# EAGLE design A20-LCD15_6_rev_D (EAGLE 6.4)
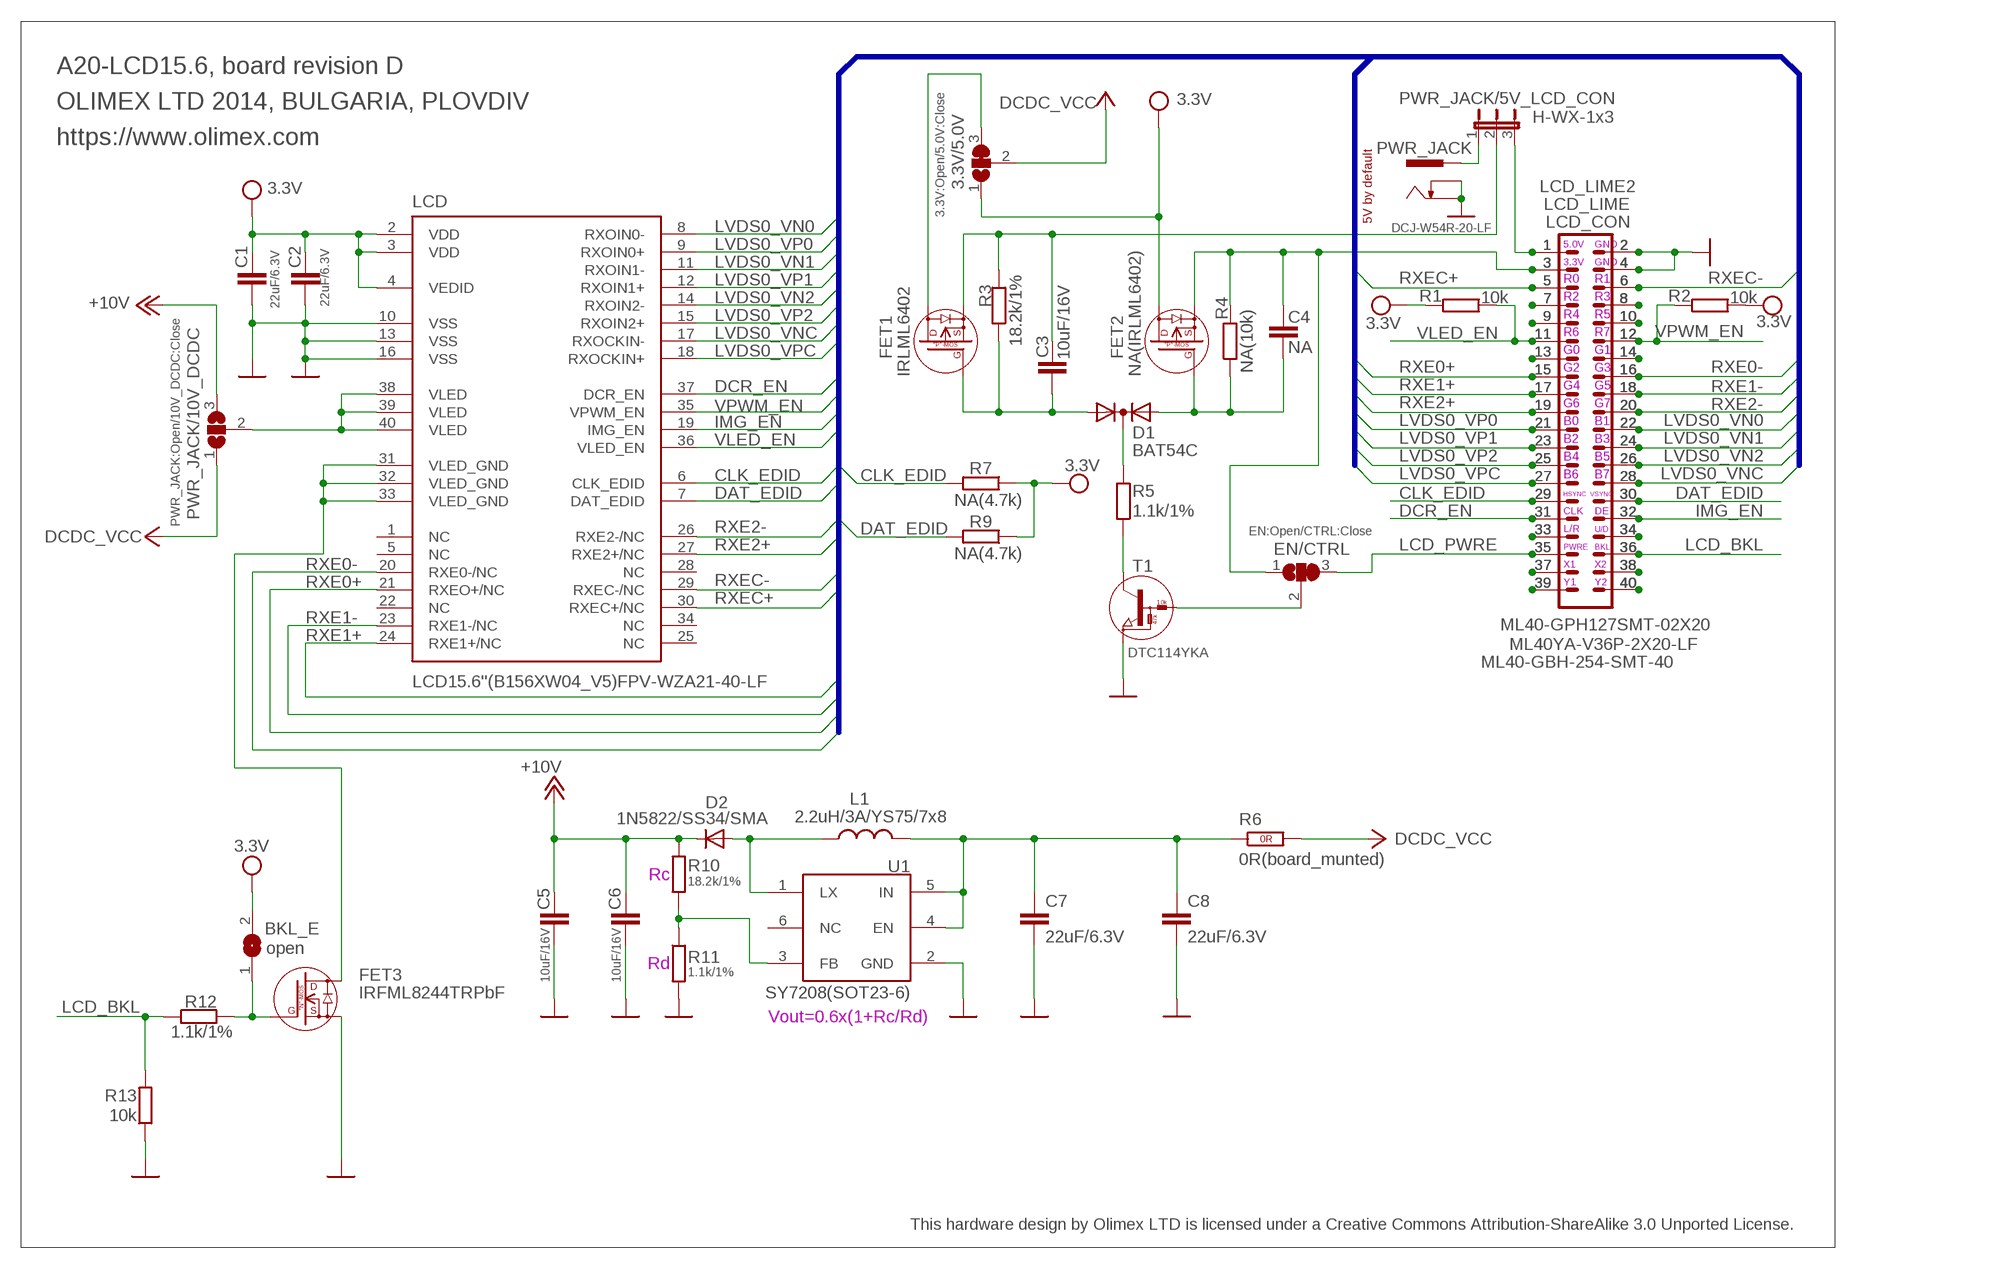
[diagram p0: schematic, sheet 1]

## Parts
3.3V/5.0V  3.3V:Open/5.0V:Close  SJ2W5  [SJ_2_SMALL_23_TIED]
BKL_E  open  SJSJ_1_THE_SMALLEST  [SJ_1_THE_SMALLEST]
C1  22uF/6.3V  C-EUC0603_DWS  [C0603_DWS]
C2  22uF/6.3V  C-EUC0603_DWS  [C0603_DWS]
C3  10uF/16V  C-EUC0805_5MIL_DWS  [C0805_5MIL_DWS]
C4  NA  C-EUC0603_DWS  [C0603_DWS]
C5  10uF/16V  C-EUC0805_5MIL_DWS  [C0805_5MIL_DWS]
C6  10uF/16V  C-EUC0805_5MIL_DWS  [C0805_5MIL_DWS]
C7  22uF/6.3V  C-EUC0805_5MIL_DWS  [C0805_5MIL_DWS]
C8  22uF/6.3V  C-EUC0805_5MIL_DWS  [C0805_5MIL_DWS]
D1  BAT54C  DIODE_AC-CA_  [SOT23C]
D2  1N5822/SS34/SMA  D-MLL-41  [MELF-MLL41]
EN/CTRL  EN:Open/CTRL:Close  SJ2W5  [SJ_2_SMALL_23_TIED]
FET1  IRLML6402  P-MOS+DIODIRLML6402  [SOT23]
FET2  NA(IRLML6402)  P-MOS+DIODIRLML6402  [SOT23]
FET3  IRFML8244TRPbF  N-MOS+DIODBSS138(SOT23-3)  [SOT23]
L1  2.2uH/3A/YS75/7x8  LLQH88PN100M38  [8X8MM_3131]
LCD  LCD15.6''(B156XW04_V5)FPV-WZA21-40-LF  [LCD_15.6'']
LCD_CON  ML40-GBH-254-SMT-40  [ML40-MALE(GBH-254-SMT-40)]
LCD_LIME  ML40YA-V36P-2X20-LF  [YA-V36P-2X20-LF]
LCD_LIME2  ML40-GPH127SMT-02X20  ML40-GPH127SMT-02X20(PA-V16X-2X20-LF)  [GPH127SMT-02X20(PA-V16X-2X20-LF)]
PWR_JACK  DCJ-W54R-20-LF  PWR-JAKDCJ-W  [PWR-JACK-SMD]
PWR_JACK/5V_LCD_CON  H-WX-1x3  JP2EHN1X3-SMD  [HN1X3-SMD]
PWR_JACK/10V_DCDC  PWR_JACK:Open/10V_DCDC:Close  SJ2W3  [SJ_2_SMALL]
R1  10k  R-EU_R0603_5MIL_DWS  [R0603_5MIL_DWS]
R2  10k  R-EU_R0603_5MIL_DWS  [R0603_5MIL_DWS]
R3  18.2k/1%  R-EU_R0603_5MIL_DWS  [R0603_5MIL_DWS]
R4  NA(10k)  R-EU_R0603_5MIL_DWS  [R0603_5MIL_DWS]
R5  1.1k/1%  R-EU_R0603_5MIL_DWS  [R0603_5MIL_DWS]
R6  0R(board_munted)  R_0R0R(NA)  [0603_0R]
R7  NA(4.7k)  R-EU_R0603_5MIL_DWS  [R0603_5MIL_DWS]
R9  NA(4.7k)  R-EU_R0603_5MIL_DWS  [R0603_5MIL_DWS]
R10  18.2k/1%  R-EU_R0603_5MIL_DWS  [R0603_5MIL_DWS]
R11  1.1k/1%  R-EU_R0603_5MIL_DWS  [R0603_5MIL_DWS]
R12  1.1k/1%  R-EU_R0603_5MIL_DWS  [R0603_5MIL_DWS]
R13  10k  R-EU_R0603_5MIL_DWS  [R0603_5MIL_DWS]
T1  DTC114YKA  DIGITAL_TRANSISTORS-NPNDTC114YKA  [SOT-23]
U1  SY7208(SOT23-6)  SY7208  [SOT23-6]

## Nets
3.3VDC [pwr]: C4.1 EN/CTRL.1 FET2.2(S) LCD_CON.3 LCD_LIME2.3 LCD_LIME.3 R4.2
5VDC: C3.1 FET1.2(S) PWR_JACK/5V_LCD_CON.2 R3.2
+5V: 3.3V/5.0V.2 PWR_JACK/10V_DCDC.1 R6.2(1.2) ; supply symbol labelled DCDC_VCC
+12V [pwr]: C5.1 C6.1 D2.1(C) PWR_JACK/10V_DCDC.3 R10.2 ; supply symbol labelled +10V
CLK_EDID: LCD.6(CLK_EDID) LCD_CON.29 LCD_LIME2.29 LCD_LIME.29 R7.2
DAT_EDID: LCD.7(DAT_EDID) LCD_CON.30 LCD_LIME2.30 LCD_LIME.30 R9.2
DCR_EN: LCD.37(DCR_EN) LCD_CON.31 LCD_LIME2.31 LCD_LIME.31
GND [pwr]: C1.2 C2.2 C5.2 C6.2 C7.2 C8.2 FET3.2(S) LCD.10(VSS) LCD.13(VSS) LCD.16(VSS) LCD_CON.2 LCD_CON.4 LCD_LIME2.2 LCD_LIME2.4 LCD_LIME.2 LCD_LIME.4 PWR_JACK.2(-) PWR_JACK.3(--) R11.2 R13.1 T1.2(E) U1.2(GND)
IMG_EN: LCD.19(IMG_EN) LCD_CON.32 LCD_LIME2.32 LCD_LIME.32
LCD_BKL: LCD_CON.36 LCD_LIME2.36 LCD_LIME.36 R12.1 R13.2
LCD_PWRE: EN/CTRL.3 LCD_CON.35 LCD_LIME2.35 LCD_LIME.35
LVDS0_VN0: LCD.8(RXOIN0-) LCD_CON.22 LCD_LIME2.22 LCD_LIME.22
LVDS0_VN1: LCD.11(RXOIN1-) LCD_CON.24 LCD_LIME2.24 LCD_LIME.24
LVDS0_VN2: LCD.14(RXOIN2-) LCD_CON.26 LCD_LIME2.26 LCD_LIME.26
LVDS0_VNC: LCD.17(RXOCKIN-) LCD_CON.28 LCD_LIME2.28 LCD_LIME.28
LVDS0_VP0: LCD.9(RXOIN0+) LCD_CON.21 LCD_LIME2.21 LCD_LIME.21
LVDS0_VP1: LCD.12(RXOIN1+) LCD_CON.23 LCD_LIME2.23 LCD_LIME.23
LVDS0_VP2: LCD.15(RXOIN2+) LCD_CON.25 LCD_LIME2.25 LCD_LIME.25
LVDS0_VPC: LCD.18(RXOCKIN+) LCD_CON.27 LCD_LIME2.27 LCD_LIME.27
N$1: 3.3V/5.0V.3 FET1.3(D)
N$2 [pwr]: FET3.3(D) LCD.31(VLED_GND) LCD.32(VLED_GND) LCD.33(VLED_GND)
N$3 [pwr]: LCD.38(VLED) LCD.39(VLED) LCD.40(VLED) PWR_JACK/10V_DCDC.2
N$4: BKL_E.1 FET3.1(G) R12.2
N$5: LCD_CON.7 LCD_LIME2.7 LCD_LIME.7
N$6: LCD_CON.9 LCD_LIME2.9 LCD_LIME.9
N$7: LCD_CON.13 LCD_LIME2.13 LCD_LIME.13
N$8: C4.2 D1.1(A1) FET2.1(G) R4.1
N$9: C3.2 D1.2(A2) FET1.1(G) R3.1
N$10: LCD_CON.33 LCD_LIME2.33 LCD_LIME.33
N$11: R5.1 T1.3(C)
N$12: LCD_CON.37 LCD_LIME2.37 LCD_LIME.37
N$13: LCD_CON.39 LCD_LIME2.39 LCD_LIME.39
N$14: LCD_CON.8 LCD_LIME2.8 LCD_LIME.8
N$15: LCD_CON.10 LCD_LIME2.10 LCD_LIME.10
N$16: EN/CTRL.2 T1.1(B)
N$17: LCD_CON.14 LCD_LIME2.14 LCD_LIME.14
N$18: LCD_CON.34 LCD_LIME2.34 LCD_LIME.34
N$19: D1.3(K) R5.2
N$20: LCD_CON.1 LCD_LIME2.1 LCD_LIME.1 PWR_JACK/5V_LCD_CON.3
N$21: LCD_CON.38 LCD_LIME2.38 LCD_LIME.38
N$22 [pwr]: PWR_JACK.1(+) PWR_JACK/5V_LCD_CON.1
N$23: LCD_CON.40 LCD_LIME2.40 LCD_LIME.40
N$24: C7.1 C8.1 L1.2 R6.1(1.1) U1.4(EN) U1.5(IN)
N$123: D2.2(A) L1.1 U1.1(LX)
N$126: R10.1 R11.1 U1.3(FB)
RXE0+: LCD.21(RXEO+/NC) LCD_CON.15 LCD_LIME2.15 LCD_LIME.15
RXE0-: LCD.20(RXE0-/NC) LCD_CON.16 LCD_LIME2.16 LCD_LIME.16
RXE1+: LCD.24(RXE1+/NC) LCD_CON.17 LCD_LIME2.17 LCD_LIME.17
RXE1-: LCD.23(RXE1-/NC) LCD_CON.18 LCD_LIME2.18 LCD_LIME.18
RXE2+: LCD.27(RXE2+/NC) LCD_CON.19 LCD_LIME2.19 LCD_LIME.19
RXE2-: LCD.26(RXE2-/NC) LCD_CON.20 LCD_LIME2.20 LCD_LIME.20
RXEC+: LCD.30(RXEC+/NC) LCD_CON.5 LCD_LIME2.5 LCD_LIME.5
RXEC-: LCD.29(RXEC-/NC) LCD_CON.6 LCD_LIME2.6 LCD_LIME.6
VCC [pwr]: 3.3V/5.0V.1 BKL_E.2 C1.1 C2.1 FET2.3(D) LCD.2(VDD) LCD.3(VDD) LCD.4(VEDID) R1.2 R2.1 R7.1 R9.1 ; supply symbol labelled 3.3V
VLED_EN: LCD.36(VLED_EN) LCD_CON.11 LCD_LIME2.11 LCD_LIME.11 R1.1
VPWM_EN: LCD.35(VPWM_EN) LCD_CON.12 LCD_LIME2.12 LCD_LIME.12 R2.2
Unconnected: LCD.1(NC) LCD.5(NC) LCD.22(NC) LCD.25(NC) LCD.28(NC) LCD.34(NC) U1.6(NC)

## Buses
LVDS0_VP[0..2],LVDS0_VN[0..2],LVDS0_VPC,LVDS0_VNC,CLK_EDID,DAT_EDID,DCR_EN,IMG_EN,VPWM_EN,VLED_EN,RXE0-,RXE0+,RXE1-,RXE1+,RXE2-,RXE2+,RXEC-,RXEC+

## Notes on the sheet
- A20-LCD15.6, board revision D
- OLIMEX LTD 2014, BULGARIA, PLOVDIV
- https://www.olimex.com
- 5V by default
- 5.0V | GND
- 3.3V | GND
- R0 | R1
- R2 | R3
- R4 | R5
- R6 | R7
- G0 | G1
- G2 | G3
- G4 | G5
- G6 | G7
- B0 | B1
- B2 | B3
- B4 | B5
- B6 | B7
- HSYNC | VSYNC
- CLK | DE
- L/R | U/D
- PWRE | BKL
- X1 | X2
- Y1 | Y2
- Rc
- Rd
- Vout=0.6x(1+Rc/Rd)
- This hardware design by Olimex LTD is licensed under a Creative Commons Attribution-ShareAlike 3.0 Unported License.

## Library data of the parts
3.3V/5.0V EN/CTRL PWR_JACK/10V_DCDC = jumper:SJ2W: SMD solder JUMPER
BKL_E = jumper:SJ: SMD solder JUMPER
C1-C8 = rcl:C-EU: CAPACITOR, European symbol
D1 = semicon-smd-ipc:DIODE_AC-CA_: DUAL DIODE
D2 = semicon-smd-ipc:D-: DIODE
FET1 FET2 = Penko:P-MOS+DIOD
FET3 = Penko:N-MOS+DIOD
L1 = OLIMEX_DISCRET:L
LCD = olimex_lcd:LCD15.6''(B156XW04_V5): LCD B156XW04 V5 LCD type: Color Active Matrix Liquid Cristal Display composed of a TFT LCD panel, a driver circuit, and LED backlight system Screen format: 16x9 HD(1366x768 pixels) Number of colors: 262K colors(RGB 6-bits data driver) Pixel Pitch: 0.252x0.252mm Pixel Format: RGB Vertical Stripe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
LCD_CON LCD_LIME LCD_LIME2 = con-harting-ml:ML40: HARTING
PWR_JACK = gogo:PWR-JAK
PWR_JACK/5V_LCD_CON = jumper:JP2E: JUMPER
R1-R5 R7 R9-R13 = rcl:R-EU_: RESISTOR, European symbol
R6 = OLIMEX_DISCRET:R_0R
T1 = OLIMEX_DISCRET:DIGITAL_TRANSISTORS-NPN: DTC114YKA Digital Transistor - NPN
U1 = OLIMEX_IC:SY7208

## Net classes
1 pwr: width 0.254 mm, drill 0.254 mm, clearance 0.241 mm

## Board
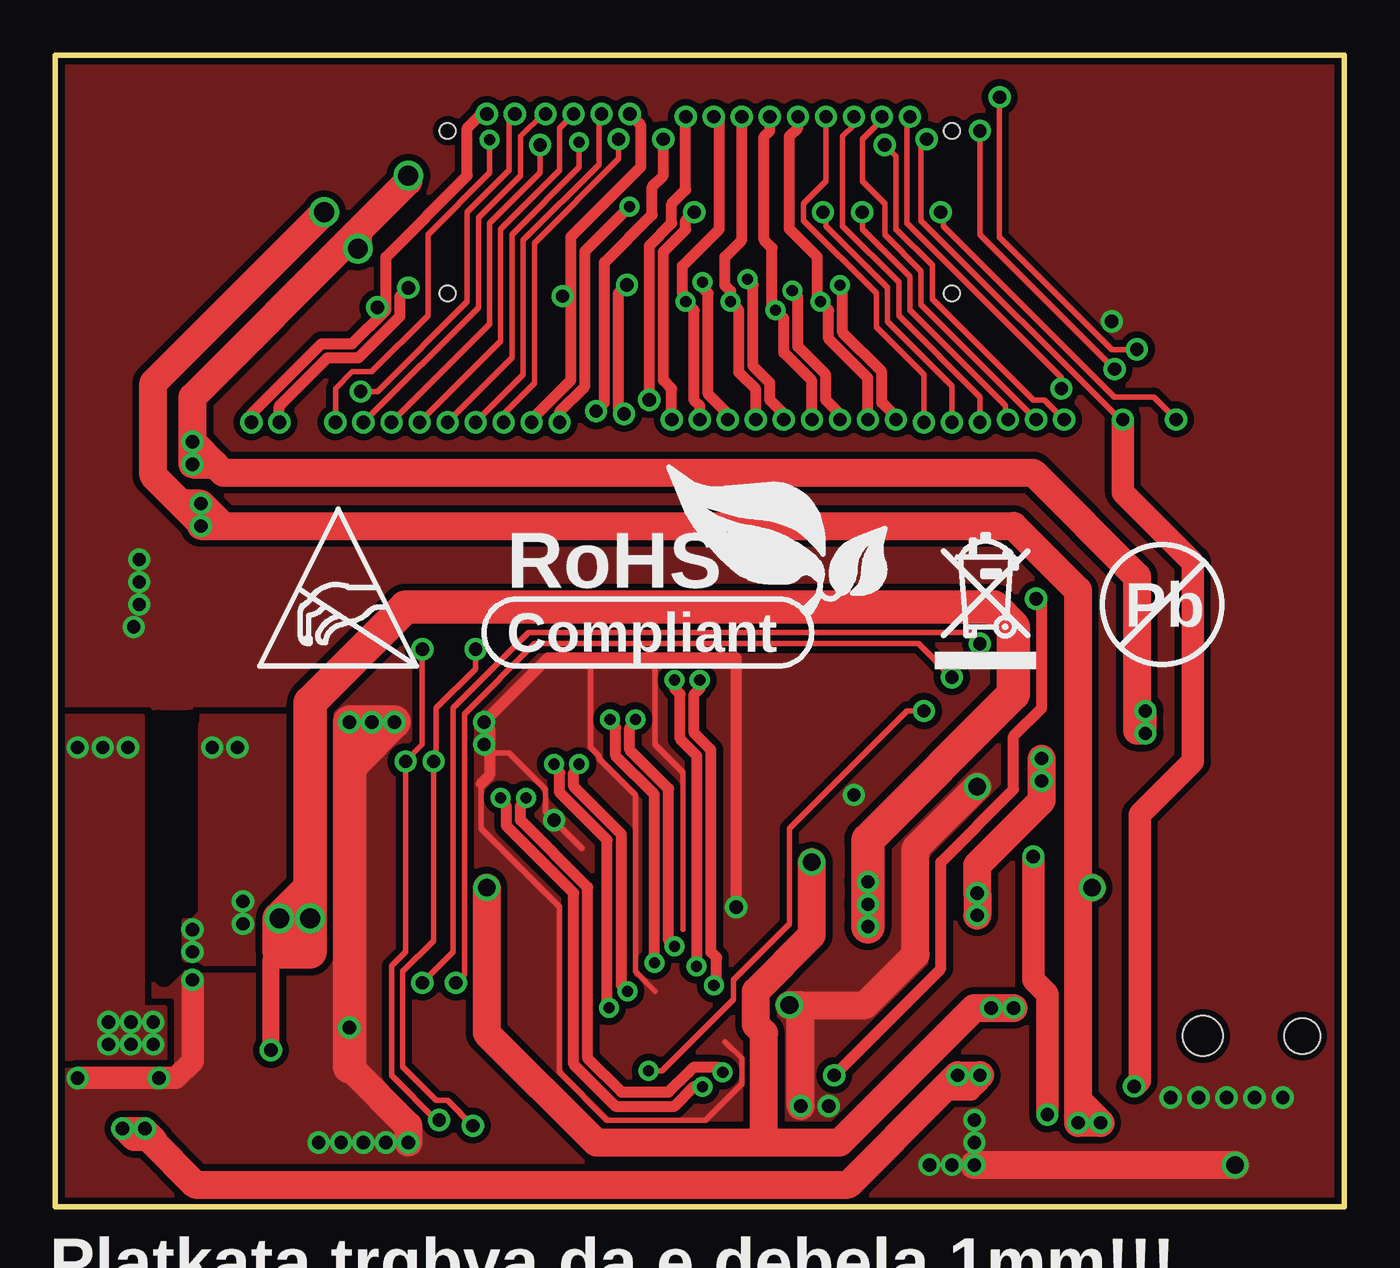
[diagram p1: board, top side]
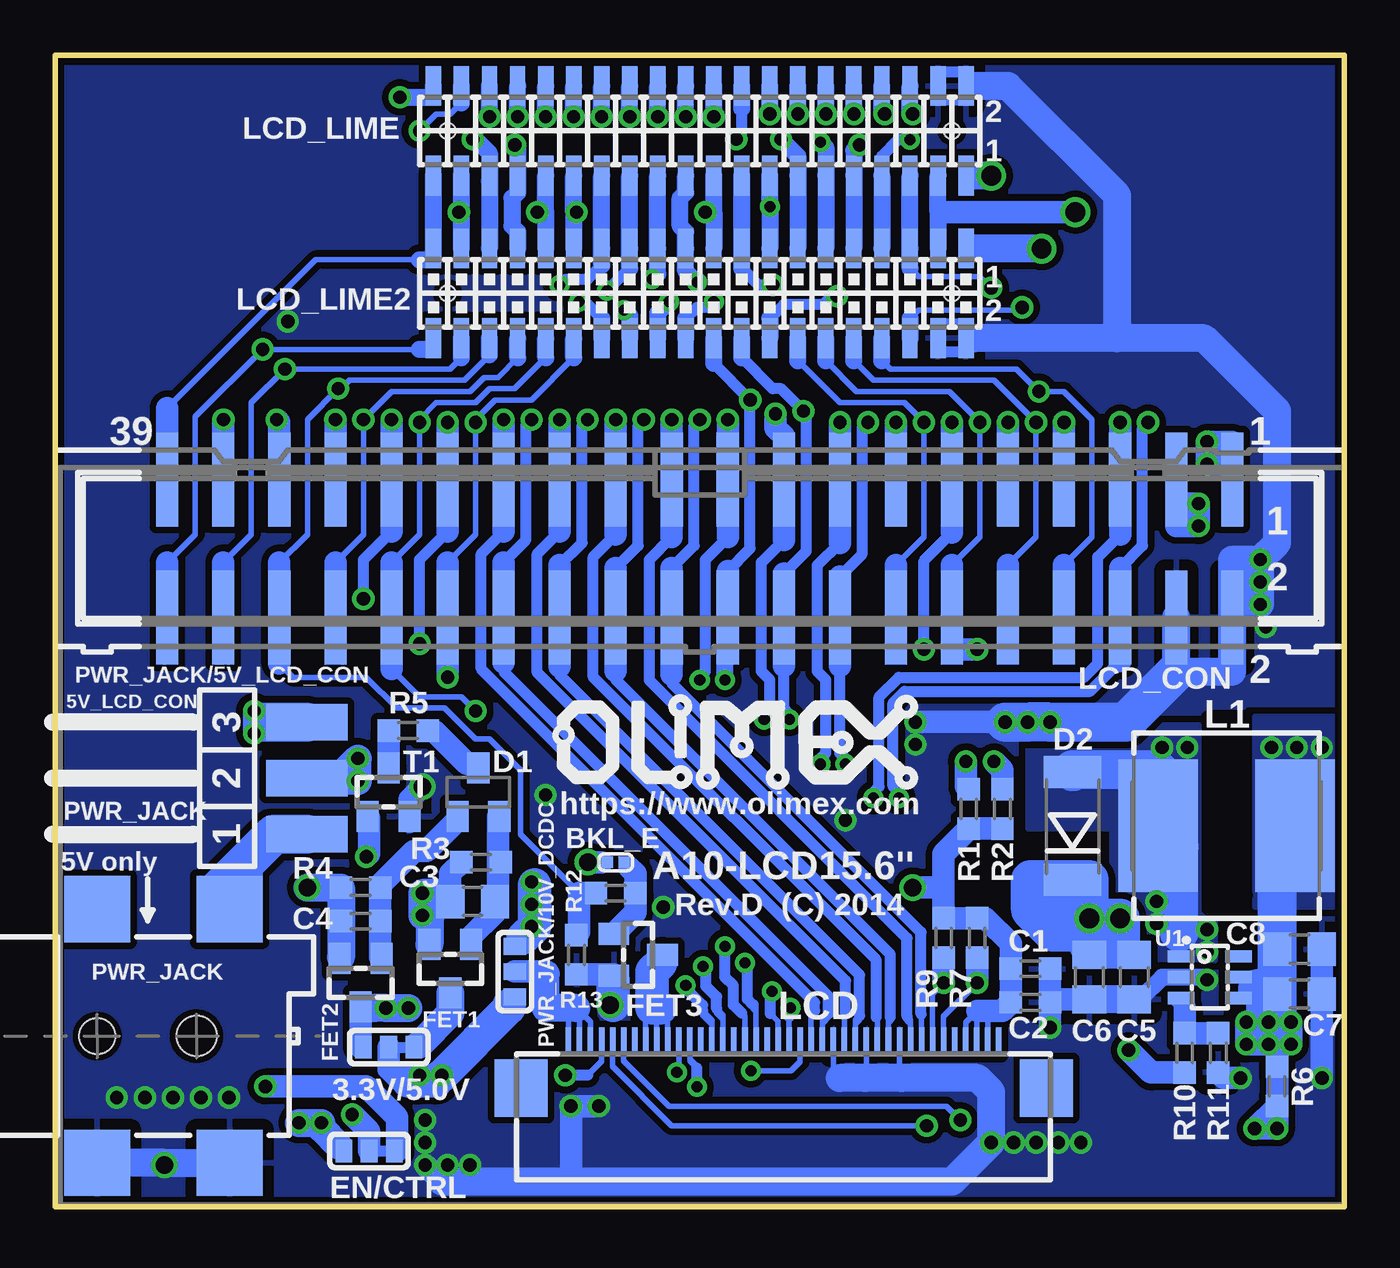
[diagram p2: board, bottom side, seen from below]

Size 58.42 x 52.2 mm. Coordinates in mm from the lower left corner, seen from the top.
Outline: 0,52.2 0,0 58.42,0 58.42,52.2 0,52.2
Copper layers (1+16): Top 0.035mm / dielectric 1mm / Bottom 0.035mm
Design rules "default": minimum track width 9.5mil, minimum drill 0.5mm, track to track 5mil, track to pad 8mil, pad to pad 8mil, via to via 8mil, smd to smd 1mil, copper to edge 10mil, drill to drill 8mil, minimum pad ring 8mil, minimum via ring 8mil, stop-mask expansion 4mil, vias tented up to drill 40mil, thermal gap 20mil
tRestrict: 3 lines
bRestrict: 2 lines

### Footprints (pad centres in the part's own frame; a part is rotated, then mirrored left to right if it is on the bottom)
SJ_2_SMALL_23_TIED = smd 0.762 x 1.016: 1 -1.143,0; 2 0,0; 3 1.143,0
SJ_1_THE_SMALLEST = smd 0.508 x 0.508: 1 -0.381,0; 2 0.381,0
C0603_DWS = smd 1.016 x 1.016: 1 -0.889,0; 2 0.889,0
C0805_5MIL_DWS = smd 1.27 x 1.524: 1 -1.016,0; 2 1.016,0
SOT23C = smd 1 x 1.4: 1 -0.95,-1.1; 2 0.95,-1.1; 3 0,1.1
MELF-MLL41 = smd 1.45 x 2.6: 1 -2.445,0; 2 2.445,0
SOT23 = smd 1 x 1.4: 1 -0.95,-1.1; 2 0.95,-1.1; 3 0,1.1
8X8MM_3131 = smd 3.6 x 6: 1 -3.1,0; 2 3.1,0
LCD_15.6'' = smd 0.25 x 1.3 bottom: 1 -67.54,31.89; 2 -67.04,31.89; 3 -66.54,31.89; 4 -66.04,31.89; 5 -65.54,31.89; 6 -65.04,31.89; 7 -64.54,31.89; 8 -64.04,31.89; 9 -63.54,31.89; 10 -63.04,31.89; 11 -62.54,31.89; 12 -62.04,31.89; 13 -61.54,31.89; 14 -61.04,31.89; 15 -60.54,31.89; 16 -60.04,31.89; 17 -59.54,31.89; 18 -59.04,31.89; 19 -58.54,31.89; 20 -58.04,31.89; 21 -57.54,31.89; 22 -57.04,31.89; 23 -56.54,31.89; 24 -56.04,31.89; 25 -55.54,31.89; 26 -55.04,31.89; 27 -54.54,31.89; 28 -54.04,31.89; 29 -53.54,31.89; 30 -53.04,31.89; 31 -52.54,31.89; 32 -52.04,31.89; 33 -51.54,31.89; 34 -51.04,31.89; 35 -50.54,31.89; 36 -50.04,31.89; 37 -49.54,31.89; 38 -49.04,31.89; 39 -48.54,31.89; 40 -48.04,31.89 | smd 2.4 x 2.6 bottom: P1 -69.69,29.79; P2 -45.89,29.79
ML40-MALE(GBH-254-SMT-40) = smd 1 x 4.25: 1 -24.13,-3.125; 2 -24.13,3.125; 3 -21.59,-3.125; 4 -21.59,3.125; 5 -19.05,-3.125; 6 -19.05,3.125; 7 -16.51,-3.125; 8 -16.51,3.125; 9 -13.97,-3.125; 10 -13.97,3.125; 11 -11.43,-3.125; 12 -11.43,3.125; 13 -8.89,-3.125; 14 -8.89,3.125; 15 -6.35,-3.125; 16 -6.35,3.125; 17 -3.81,-3.125; 18 -3.81,3.125; 19 -1.27,-3.125; 20 -1.27,3.125; 21 1.27,-3.125; 22 1.27,3.125; 23 3.81,-3.125; 24 3.81,3.125; 25 6.35,-3.125; 26 6.35,3.125; 27 8.89,-3.125; 28 8.89,3.125; 29 11.43,-3.125; 30 11.43,3.125; 31 13.97,-3.125; 32 13.97,3.125; 33 16.51,-3.125; 34 16.51,3.125; 35 19.05,-3.125; 36 19.05,3.125; 37 21.59,-3.125; 38 21.59,3.125; 39 24.13,-3.125; 40 24.13,3.125
YA-V36P-2X20-LF = smd 0.7 x 1.8: 1 -12.065,2.032; 2 -12.065,-2.032; 3 -10.795,2.032; 4 -10.795,-2.032; 5 -9.525,2.032; 6 -9.525,-2.032; 7 -8.255,2.032; 8 -8.255,-2.032; 9 -6.985,2.032; 10 -6.985,-2.032; 11 -5.715,2.032; 12 -5.715,-2.032; 13 -4.445,2.032; 14 -4.445,-2.032; 15 -3.175,2.032; 16 -3.175,-2.032; 17 -1.905,2.032; 18 -1.905,-2.032; 19 -0.635,2.032; 20 -0.635,-2.032; 21 0.635,2.032; 22 0.635,-2.032; 23 1.905,2.032; 24 1.905,-2.032; 25 3.175,2.032; 26 3.175,-2.032; 27 4.445,2.032; 28 4.445,-2.032; 29 5.715,2.032; 30 5.715,-2.032; 31 6.985,2.032; 32 6.985,-2.032; 33 8.255,2.032; 34 8.255,-2.032; 35 9.525,2.032; 36 9.525,-2.032; 37 10.795,2.032; 38 10.795,-2.032; 39 12.065,2.032; 40 12.065,-2.032 | hole 0.7: -11.43,0; 11.43,0
GPH127SMT-02X20(PA-V16X-2X20-LF) = smd 0.7 x 1.8: 1 -12.065,-2.032; 2 -12.065,2.032; 3 -10.795,-2.032; 4 -10.795,2.032; 5 -9.525,-2.032; 6 -9.525,2.032; 7 -8.255,-2.032; 8 -8.255,2.032; 9 -6.985,-2.032; 10 -6.985,2.032; 11 -5.715,-2.032; 12 -5.715,2.032; 13 -4.445,-2.032; 14 -4.445,2.032; 15 -3.175,-2.032; 16 -3.175,2.032; 17 -1.905,-2.032; 18 -1.905,2.032; 19 -0.635,-2.032; 20 -0.635,2.032; 21 0.635,-2.032; 22 0.635,2.032; 23 1.905,-2.032; 24 1.905,2.032; 25 3.175,-2.032; 26 3.175,2.032; 27 4.445,-2.032; 28 4.445,2.032; 29 5.715,-2.032; 30 5.715,2.032; 31 6.985,-2.032; 32 6.985,2.032; 33 8.255,-2.032; 34 8.255,2.032; 35 9.525,-2.032; 36 9.525,2.032; 37 10.795,-2.032; 38 10.795,2.032; 39 12.065,-2.032; 40 12.065,2.032 | hole 0.7: -11.43,0; 11.43,0
PWR-JACK-SMD = smd 3 x 3: 1 6,5.75; 2 0,-5.75; 3 6,-5.75; 4 0,5.75 | hole 1.6: 0,0 | hole 1.8: 4.5,0
HN1X3-SMD = smd 1.651 x 3.683: 1 -2.54,-0.229; 2 0,-0.229; 3 2.54,-0.229
SJ_2_SMALL = smd 0.762 x 1.016: 1 -1.143,0; 2 0,0; 3 1.143,0
R0603_5MIL_DWS = smd 1.016 x 1.016: 1 -0.889,0; 2 0.889,0
0603_0R = smd 1.016 x 1.016: 1 -0.889,0; 2 0.889,0
SOT-23 = smd 1 x 1.4: 1 -0.95,-1.1; 2 0.95,-1.1; 3 0,1.1
SOT23-6 = smd 0.55 x 1.2: 1 -0.95,-1.3; 2 0,-1.3; 3 0.95,-1.3; 4 0.95,1.3; 5 0,1.3; 6 -0.95,1.3

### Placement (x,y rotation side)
3.3V/5.0V  43.31,7.24 0 bottom
BKL_E  33.02,15.62 180 bottom
C1  14.22,10.79 0 bottom
C2  14.22,9.27 0 bottom
C3  39.5,13.84 0 bottom
C4  44.58,12.95 0 bottom
C5  9.53,10.41 270 bottom
C6  11.56,10.41 270 bottom
C7  2.03,9.65 0 bottom
C8  2.03,11.68 0 bottom
D1  39.24,18.8 0 bottom
D2  12.32,17.27 90 bottom
EN/CTRL  44.2,2.54 0 bottom
FET1  40.51,10.79 180 bottom
FET2  44.58,10.16 180 bottom
FET3  32,11.43 270 bottom
L1  5.33,17.27 0 bottom
LCD  83.2,-24.4 0 top
LCD_CON  29.21,29.84 180 bottom
LCD_LIME  29.21,48.77 180 bottom
LCD_LIME2  29.21,41.4 180 bottom
PWR_JACK  56.52,7.75 0 bottom
PWR_JACK/5V_LCD_CON  47.24,19.43 90 bottom
PWR_JACK/10V_DCDC  37.59,10.67 90 bottom
R1  17.02,18.03 270 bottom
R2  15.49,18.03 90 bottom
R3  39.12,15.62 180 bottom
R4  44.58,14.48 180 bottom
R5  42.42,21.59 0 bottom
R6  3.05,5.46 270 bottom
R7  16.64,12.19 270 bottom
R9  18.16,12.19 270 bottom
R10  7.24,6.99 270 bottom
R11  5.71,6.99 270 bottom
R12  33.02,14.22 0 bottom
R13  34.8,11.43 90 bottom
T1  43.31,18.8 0 bottom
U1  6.1,10.41 270 bottom
U$5  [ROHS]  20.45,25.15 0 top
U$6  [PB]  50.16,27.3 0 top
U$8  [OLIMEX1_V]  18.16,18.8 0 bottom
U$10  [ESD_SYMBOL]  9.27,24.51 0 top
U$11  [RECYCLE_BIN1/8]  39.88,24.38 0 top

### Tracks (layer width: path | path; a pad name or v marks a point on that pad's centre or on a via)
3.3VDC  (via drill 0.6, 0.8, 0.9)
  Top 1.27: 7.62,30.86 v6.6,31.88 | v6.6,30.86 7.62,30.86 | v6.6,30.86 v6.6,31.88 | 7.62,30.86 43.43,30.86 46.35,27.94 46.35,14.48 | 46.35,14.48 46.35,4.83 | 46.35,4.83 v47.37,3.81 v46.35,3.81 46.35,4.83 | 46.35,14.48 v46.99,14.48 | v6.6,31.88 5.71,31.88 | 5.71,31.88 4.45,33.15 4.45,37.34 v12.19,45.09 | v6.6,30.86 6.6,30.99 5.71,31.88
  Bottom 0.508: 18.16,45.09 18.41,45.09
  Bottom 0.762: 45.59,2.79 EN/CTRL.1 | LCD_LIME2.3 18.41,45.09 LCD_LIME.3
  Bottom 1.016: 7.62,31.88 LCD_CON.3 | 7.62,31.88 v6.6,31.88 v6.6,30.86 7.62,30.86 7.62,31.88 | 45.47,11.32 FET2.2 | v12.19,45.09 18.16,45.09
  Bottom 1.27: 45.47,11.32 C4.1 R4.2 v46.99,14.48 | 45.59,2.79 46.35,3.56 v46.35,3.81 v47.37,3.81
5VDC  (via drill 0.6)
  Top 1.27: v44.7,20.32 v44.7,19.3 44.7,18.41 41.78,15.49 v41.78,14.22 v41.78,13.21
  Bottom 1.016: 40.51,14.22 40.51,15.11 R3.2
  Bottom 1.27: 45.72,19.3 v44.7,19.3 v44.7,20.32 45.72,19.3 | 45.72,19.3 46.89,19.3 PWR_JACK/5V_LCD_CON.2 | 41.46,13.21 FET1.2 | 41.46,13.21 41.4,13.21 | 41.46,13.21 v41.78,13.21 v41.78,14.22 40.51,14.22 C3.1
+5V  (via drill 0.6)
  Top 0.762: v41.91,5.97 41.91,5.59 41.53,5.21 40.13,5.21
  Top 1.016: v4.06,3.56 4.57,3.05 4.32,3.05 3.56,3.05 v3.05,3.56 v4.06,3.56
  Top 1.27: v41.91,5.97 v40.89,5.97 40.13,5.21 35.94,1.02 6.35,1.02 4.32,3.05
  Bottom 0.508: PWR_JACK/10V_DCDC.1 37.59,9.4 37.85,9.14 | v41.91,5.97 41.91,5.71
  Bottom 0.762: 42.55,5.71 42.95,5.71 43.43,6.2 43.43,7.11 3.3V/5.0V.2
  Bottom 1.016: 42.42,5.71 42.55,5.71 42.67,5.71 43.31,6.35 3.3V/5.0V.2 | R6.2 v3.05,3.56 v4.06,3.56 R6.2
  Bottom 1.524: 37.85,9.14 37.85,9.02 v40.89,5.97 41.15,5.71 41.91,5.71 42.42,5.71
+12V  (via drill 0.6, 0.9)
  Top 0.762: v9.78,7.11 9.78,11.18 10.16,11.56
  Top 1.524: v11.56,13.08 11.56,14.48 | v10.16,13.08 v11.56,13.08 | v10.16,13.08 11.56,14.48 | 11.56,14.48 11.56,22.86 15.88,27.18 42.55,27.18 43.43,26.29 43.43,23.24 36.83,16.64 v36.83,14.73 v36.83,13.72 v36.83,12.7 | v11.56,13.08 11.56,11.56 10.16,11.56 v10.16,13.08
  Bottom 0.508: 37.21,12.19 PWR_JACK/10V_DCDC.3
  Bottom 1.016: R10.2 8.76,6.1 v9.78,7.11 | v36.83,14.73 36.7,14.61
  Bottom 1.27: 10.16,11.43 C5.1 | 10.16,11.43 C6.1 11.56,11.81 | 10.16,12.06 10.16,11.43
  Bottom 1.524: 37.21,12.19 36.7,12.7 36.7,14.61
  Bottom 1.778: 11.56,12.45 11.56,11.81 | v11.56,13.08 11.56,12.45 | v11.56,13.08 v10.16,13.08 10.16,12.06 | v11.56,13.08 11.56,14.83 D2.1 13.21,14.83 | 13.21,12.45 13.21,14.83 | 11.56,12.45 13.21,12.45 | 13.21,12.45 14.22,13.46 14.22,14.83 13.21,14.83
CLK_EDID  (via drill 0.6)
  Top 0.254: v16.64,10.16 18.03,11.56 18.03,22.61 21.46,26.04 41.4,26.04 v41.91,25.53 | v40.64,35.56 40.64,37.21 37.72,40.13 37.72,41.66 34.92,44.45 34.92,44.96 v34.8,45.09
  Bottom 0.254: LCD.6 18.16,8.64 v16.64,10.16
  Bottom 0.508: v41.91,25.53 41.91,29.34 40.64,30.61
  Bottom 0.762: 34.92,45.09 LCD_LIME2.29 | v34.8,45.09 34.92,45.09 | 34.92,45.09 LCD_LIME.29
  Bottom 1.016: 40.64,30.61 LCD_CON.29 v40.64,35.56 | v16.64,10.16 R7.2
DAT_EDID  (via drill 0.6)
  Top 0.254: v18.16,10.16 18.54,10.54 18.54,22.35 21.72,25.53 39.12,25.53 v40.64,24 | v39.37,35.56 39.37,37.72 37.21,39.88 37.21,41.4 33.91,44.7 33.91,45.47 34.92,46.48 v34.92,49.4
  Bottom 0.254: LCD.7 18.66,9.66 v18.16,10.16 | 40.64,29.21 39.37,30.48 v39.37,35.56 39.37,35.69 38.48,36.58 36.83,36.58 34.92,38.48
  Bottom 0.762: 34.92,38.48 LCD_LIME2.30 | v34.92,49.4 LCD_LIME.30
  Bottom 1.016: v40.64,24 LCD_CON.30 40.64,29.21 | v18.16,10.16 R9.2
DCR_EN  (via drill 0.6)
  Top 0.254: v43.18,35.69 43.05,35.81 43.05,36.32 38.73,40.64 38.73,42.16 36.58,44.32 v36.58,45.09
  Top 0.508: v35.31,5.97 40.13,10.79 40.13,15.62 43.43,18.92 43.43,21.34 44.7,22.61 44.7,27.3 v44.45,27.56
  Bottom 0.254: LCD.37 33.66,6.6 34.29,5.97
  Bottom 0.508: v44.45,27.56 44.45,29.34 43.18,30.61 | 34.29,5.97 v35.31,5.97
  Bottom 0.762: 36.2,45.09 LCD_LIME2.31 | 36.2,45.09 LCD_LIME.31 | v36.58,45.09 36.2,45.09
  Bottom 1.016: 43.18,30.61 LCD_CON.31 v43.18,35.69
GND  (via drill 0.6, 0.8)
  Top 0.254: 19.3,19.18 19.3,17.14 22.86,13.59 22.86,6.1 25.02,3.94 29.46,3.94 31.11,5.59 31.11,6.73 30.35,7.49 | 24.26,24.89 24.26,20.83 24.64,20.45 24.64,20.32 26.29,18.67 26.29,10.67 27.18,9.78 | 19.68,20.57 20.57,20.57 22.23,18.92 22.23,17.91 v22.61,17.53 23.88,16.26 | 27.18,24.89 27.18,20.95 28.45,19.68 28.45,12.57
  Top 0.508: 19.3,19.18 19.68,19.56 19.68,20.57 19.68,21.72 v19.43,21.97 22.35,24.89 24.26,24.89 27.18,24.89 30.86,24.89 v30.86,13.59
  Top 1.016: v6.22,10.29 6.22,6.6 5.46,5.84 v4.7,5.84 v1.02,5.84
  Top 1.27: 13.34,6.35 16,3.68 v16,2.92 | v41.78,19.05 38.99,16.26 38.99,11.43 36.7,9.14 33.78,9.14 | 33.78,9.14 v33.27,9.14 | v41.66,1.91 v53.47,1.91 | v33.78,4.57 33.78,9.14
  Top 1.524: 13.34,6.35 v13.34,8.13 13.34,20.19 | 13.34,20.19 v13.34,21.97 v14.35,21.97 v15.37,21.97 13.59,20.19 13.34,20.19
  Bottom 0.254: 20.07,5.84 20.07,5.97 20.16,6.06 LCD.10 | LCD.13 21.66,5.9 21.72,5.84 | LCD.16 23.16,6.14 22.86,5.84
  Bottom 0.508: LCD_LIME2.2 17.14,38.73 18.41,38.73 LCD_LIME2.4 18.41,40.01 17.14,40.01 LCD_LIME2.2 | 16.76,39.37 LCD_LIME2.2 | LCD_LIME.2 17.14,51.44 18.41,51.44 LCD_LIME.4 18.41,50.16 17.14,50.16 LCD_LIME.2 | 16.76,50.8 LCD_LIME.2
  Bottom 0.762: C5.2 9.27,9.4 8.26,10.41 U1.2 6.35,10.41 v6.22,10.29
  Bottom 1.016: 40.89,1.14 v41.66,1.91 | 42.36,17.46 T1.2 42.36,18.48 v41.78,19.05 | v53.47,1.91 53.47,2 | v33.78,4.57 v35.05,4.57 35.05,1.14 | v13.34,8.13 C2.2 13.34,9.4 | C8.2 C7.2 v1.02,5.84 | 13.34,9.4 C1.2 | C6.2 13.34,9.4 | v15.37,21.97 v19.43,21.97 | v4.7,5.84 5.46,5.84 R11.2 | R13.1 33.16,10.54 FET3.2 33.15,10.48 33.15,10.29
  Bottom 1.27: PWR_JACK.3 53.47,2 PWR_JACK.2 | 40.89,1.14 35.05,1.14 17.78,1.14 v16,2.92 16,5.21 16.64,5.84 20.07,5.84 21.72,5.84 22.86,5.84 | LCD_CON.4 7.62,24.26 5.08,24.26 LCD_CON.2 5.08,27.3 | C5.2 C6.2 | v33.27,9.14 33.15,9.14 | 16.76,50.8 15.24,50.8 10.29,45.85 10.29,39.37 | 10.29,39.37 16.76,39.37 | 10.29,39.37 6.35,39.37 3.05,36.07 3.05,30.1 v3.81,29.34 | 5.08,27.3 5.08,29.34 v3.81,29.34 | v3.81,29.34 v3.81,27.3 5.08,27.3
  Bottom 1.524: 33.15,9.14 33.15,10.29
  Bottom 1.778: 7.62,24.26 9.91,21.97 v13.34,21.97 v14.35,21.97 v15.37,21.97
  other vias: 50.55,4.95 51.82,4.95 53.09,4.95 54.36,4.95 55.63,4.95 40.64,1.91 41.66,2.92 14.99,2.92 13.97,2.92 12.95,2.92 3.81,28.32 41.66,3.94 39.62,1.91 11.94,2.92 19.43,20.95 36.2,18.67 47.88,40.13 3.56,26.29
  pour Top (isolate 0.305, rank 2): 68.45,60.96 68.45,-5.08 -5.08,-5.08 -5.08,60.96
  pour Bottom (isolate 0.305, rank 3): -2.54,-2.54 64.26,-2.54 64.26,58.42 -2.54,58.42
IMG_EN  (via drill 0.5, 0.6)
  Top 0.254: v26.9,6.17 27.51,6.17 30.73,9.4 30.73,10.29 33.27,12.83 33.27,17.14 38.61,22.48 v39.37,22.48 | v41.91,35.56 41.91,36.7 38.23,40.39 38.23,41.91 35.69,44.45 35.69,48.51 36.2,49.02 v36.2,49.4
  Bottom 0.254: LCD.19 24.66,6.58 25.07,6.17 v26.9,6.17 | 43.18,24.38 41.91,23.11 40.01,23.11 v39.37,22.48 | 43.18,29.21 41.91,30.48 v41.91,35.56 41.91,35.69 41.15,36.45 39.37,36.45 38.73,37.08 37.59,37.08 36.2,38.48
  Bottom 0.762: 36.2,38.48 LCD_LIME2.32 | v36.2,49.4 LCD_LIME.32
  Bottom 1.016: 43.18,24.38 LCD_CON.32 43.18,29.21
LCD_BKL  (via drill 0.6)
  Top 0.254: v45.59,37.08 45.59,37.59 38.61,44.58 38.61,49.28 v38.73,49.4
  Bottom 0.254: 48.26,24.64 47.62,24 44.32,24 42.93,22.61 40.77,22.61 39.37,21.21 38.73,21.21 37.34,19.81 37.34,16.89 34.67,14.22 | 48.26,29.21 46.99,30.48 46.99,35.69 v45.59,37.08 45.47,37.08 45.09,37.47 39.88,37.47 38.73,38.61
  Bottom 0.762: v38.73,49.4 LCD_LIME.36 | 38.73,38.61 LCD_LIME2.36
  Bottom 1.016: 48.26,24.64 LCD_CON.36 48.26,29.21 | R13.2 34.67,12.45 34.67,14.22 R12.1
LCD_PWRE  (via drill 0.6)
  Top 0.254: v48.39,35.69 48.26,35.69 39.24,44.7 39.24,48.13 v39.5,48.39
  Top 1.016: v48.9,5.46 49.15,5.71 49.15,17.78 51.56,20.19 51.56,29.21 48.39,32.38 v48.39,35.69
  Bottom 0.508: 38.73,46.48 LCD_LIME.35
  Bottom 0.762: EN/CTRL.3 42.93,2.54 | LCD_LIME2.35 38.73,46.48 38.73,47.75 39.37,48.39 v39.5,48.39
  Bottom 1.016: 42.93,2.54 42.93,4.06 44.32,5.46 v48.9,5.46 | v48.39,35.69 48.26,35.56 LCD_CON.35
LVDS0_VN0  (via drill 0.5, 0.6)
  Top 0.508: v29.21,35.69 29.21,36.3 28.96,36.55 28.96,40.64 v28.57,41.02 28.57,41.27 28.42,41.43 28.42,42.65 30.1,44.32 30.1,49.15 v29.84,49.4
  Bottom 0.254: LCD.8 19.16,8.72 19.18,8.74
  Bottom 0.508: 30.48,24.13 30.48,23.75 19.18,12.45 19.18,8.74 | 30.48,28.96 29.46,29.97 29.46,35.43 v29.21,35.69 | v28.57,41.02 28.83,40.77 29.34,40.77 29.84,40.26
  Bottom 0.762: 29.84,40.26 LCD_LIME2.22 | v29.84,49.4 LCD_LIME.22
  Bottom 1.016: 30.48,24.13 LCD_CON.22 30.48,28.96
LVDS0_VN1  (via drill 0.5, 0.6)
  Top 0.508: v31.75,35.69 31.75,37.06 30.99,37.82 30.99,40.64 v30.61,41.02 30.61,41.5 30.35,41.76 30.35,43.05 31.11,43.81 v31.11,49.4
  Bottom 0.254: LCD.11 20.66,8.34 | 20.66,8.34 20.66,8.53 20.57,8.61 20.57,8.42 20.66,8.34
  Bottom 0.508: 20.57,8.61 20.57,11.46 33.02,23.9 33.02,24.28 | 33.02,28.96 32,29.97 32,35.43 v31.75,35.69
  Bottom 0.762: v30.61,41.02 31.11,40.51 LCD_LIME2.24 | v31.11,49.4 LCD_LIME.24
  Bottom 1.016: 33.02,24.28 LCD_CON.24 33.02,28.96
LVDS0_VN2  (via drill 0.5, 0.6)
  Top 0.508: v34.29,35.69 34.29,37.44 33.02,38.71 33.02,40.26 v32.64,40.64 32.49,40.79 32.49,43.46 32.13,43.81 32.13,48.51 32.38,48.77 v32.38,49.4
  Bottom 0.254: LCD.14 22.16,8.29 | 22.16,8.29 22.16,8.47 21.97,8.66 21.97,8.48 22.16,8.29
  Bottom 0.508: 35.56,24.49 35.56,24.11 21.97,10.52 21.97,8.66 | 35.56,29.08 34.54,30.1 34.54,35.43 v34.29,35.69
  Bottom 0.762: v32.64,40.64 32.38,40.39 LCD_LIME2.26 | v32.38,49.4 LCD_LIME.26
  Bottom 1.016: 35.56,24.49 LCD_CON.26 35.56,29.08
LVDS0_VNC  (via drill 0.5, 0.6)
  Top 0.508: v36.83,35.69 36.83,37.57 35.05,39.34 35.05,40.64 v34.67,41.02 34.54,41.15 34.54,43.05 33.27,44.32 33.27,48.51 33.66,48.9 v33.66,49.4
  Bottom 0.254: LCD.17 23.66,8.35 | 23.66,8.35 23.66,8.47 23.37,8.76 23.37,8.59 23.61,8.35 23.66,8.35
  Bottom 0.508: 38.1,24.66 38.1,24.27 23.37,9.54 23.37,8.76 | 38.1,29.21 37.08,30.23 37.08,35.43 v36.83,35.69 | v34.67,41.02 34.42,41.02 33.66,40.26
  Bottom 0.762: 33.66,40.26 LCD_LIME2.28 | v33.66,49.4 LCD_LIME.28
  Bottom 1.016: 38.1,24.66 LCD_CON.28 38.1,29.21
LVDS0_VP0  (via drill 0.5, 0.6)
  Top 0.508: v30.48,35.69 30.48,35.94 29.59,36.83 29.59,41.4 29.34,41.66 v29.34,41.91
  Bottom 0.254: LCD.9 19.66,8.31 | 19.66,8.31 19.66,8.48 19.81,8.64 19.81,8.46 19.66,8.31
  Bottom 0.508: 30.48,30.35 31.5,29.34 31.5,23.86 19.81,12.18 19.81,8.64
  Bottom 0.762: LCD_LIME.21 29.84,45.97 30.1,45.72 30.1,44.45 29.84,44.2 LCD_LIME2.21 29.84,42.42 v29.34,41.91
  Bottom 1.016: 30.48,30.35 LCD_CON.21 v30.48,35.69
LVDS0_VP1  (via drill 0.5, 0.6)
  Top 0.508: v33.02,35.69 33.02,35.94 32.38,36.58 32.38,37.34 31.62,38.1 31.62,41.78 v31.37,42.04
  Bottom 0.254: LCD.12 21.16,8.56 21.21,8.61
  Bottom 0.508: 33.02,30.48 34.04,29.46 34.04,24.02 21.21,11.19 21.21,8.61
  Bottom 0.762: LCD_LIME.23 LCD_LIME2.23 31.11,42.29 v31.37,42.04
  Bottom 1.016: 33.02,30.48 LCD_CON.23 v33.02,35.69
LVDS0_VP2  (via drill 0.5, 0.6)
  Top 0.508: v35.56,35.69 35.56,35.94 34.92,36.58 34.92,37.72 33.66,38.99 33.66,41.27 v33.4,41.53
  Bottom 0.254: LCD.15 22.66,8.53 | 22.66,8.53 22.66,8.71 22.61,8.76 22.61,8.58 22.66,8.53
  Bottom 0.508: 35.56,30.61 36.58,29.59 36.58,24.22 22.61,10.25 22.61,8.76 | v33.4,41.53 32.38,42.55
  Bottom 0.762: LCD_LIME.25 LCD_LIME2.25 32.38,42.55
  Bottom 1.016: 35.56,30.61 LCD_CON.25 v35.56,35.69
LVDS0_VPC  (via drill 0.5, 0.6)
  Top 0.508: v38.1,35.69 38.1,35.81 37.47,36.45 37.47,37.85 35.69,39.62 35.69,41.66 v35.56,41.78
  Bottom 0.254: LCD.18 24.16,8.56 | 24.16,8.56 24.16,8.73 24,8.89 24,8.71 24.16,8.56
  Bottom 0.508: 38.1,30.61 39.12,29.59 39.12,24.38 24,9.27 24,8.89 | v35.56,41.78 35.31,42.04 34.29,42.04 33.66,42.67
  Bottom 0.762: LCD_LIME.27 LCD_LIME2.27 33.66,42.67
  Bottom 1.016: 38.1,30.61 LCD_CON.27 v38.1,35.69
N$1
  Bottom 0.762: 41.91,7.37 42.04,7.24 3.3V/5.0V.3
  Bottom 1.27: FET1.3 40.51,8.76 41.91,7.37
N$2
  Bottom 0.254: LCD.32 31.16,8.85 30.99,9.02 30.66,8.69 LCD.31 | LCD.33 31.66,8.73 31.37,9.02
  Bottom 1.016: FET3.3 30.9,11.13 30.99,11.05
  Bottom 1.524: 30.99,9.02 31.37,9.02 31.37,10.67 30.99,11.05
N$3
  Bottom 0.254: LCD.38 34.16,8.38 34.66,8.88 | LCD.40 35.16,8.65 34.8,9.02 34.66,8.88 | LCD.39 34.66,8.88
  Bottom 1.016: 36.45,10.54 36.58,10.67 PWR_JACK/10V_DCDC.2
  Bottom 1.27: 34.8,9.02 36.2,9.02 36.2,10.54 36.45,10.54
N$4
  Bottom 0.508: 32.38,15.37 BKL_E.1
  Bottom 1.016: 32.38,15.37 32.13,15.11 R12.2 32.13,13.35 FET3.1
N$5  (via drill 0.5, 0.6)
  Top 0.254: v19.68,48.36 19.68,46.86 16.89,44.07 16.89,40.39 14.35,37.85 13.46,37.85 12.7,37.08 v12.7,35.56
  Bottom 0.508: LCD_LIME.7 20.95,47.62 20.22,48.36 v19.68,48.36
  Bottom 0.762: LCD_LIME.7 LCD_LIME2.7
  Bottom 1.016: LCD_CON.7 v12.7,35.56
N$6  (via drill 0.6)
  Top 0.254: v21.97,48.13 21.97,46.86 19.68,44.58 19.68,40.01 v15.24,35.56
  Bottom 0.762: LCD_LIME2.9 LCD_LIME.9 22.23,47.88 v21.97,48.13
  Bottom 1.016: LCD_CON.9 v15.24,35.56
N$7  (via drill 0.6)
  Top 0.254: v20.32,35.56 20.32,35.94 21.72,37.34 21.72,43.69 25.53,47.5 v25.53,48.39
  Bottom 0.762: LCD_LIME2.13 LCD_LIME.13 24.77,47.62 v25.53,48.39
  Bottom 1.016: LCD_CON.13 v20.32,35.56
N$8
  Bottom 1.016: D1.1 40.19,17.53 41.59,16.13 42.16,16.13 43.69,14.61 R4.1 C4.2 43.69,11.32 FET2.1
N$9
  Bottom 1.016: FET1.1 39.56,12.25 38.48,13.34 C3.2 38.35,13.84 38.35,15.62 | 38.35,15.62 R3.1 | D1.2 38.35,17.7 38.35,15.62
N$10  (via drill 0.6)
  Top 0.254: v45.72,35.69 44.83,36.58 44.32,36.58 39.75,41.15 39.75,42.67 38.1,44.32 38.1,47.62 v37.59,48.13
  Bottom 0.762: LCD_LIME2.33 37.47,44.2 37.72,44.45 37.72,45.72 37.47,45.97 LCD_LIME.33 37.47,48.01 v37.59,48.13
  Bottom 1.016: LCD_CON.33 v45.72,35.69
N$11
  Bottom 1.016: T1.3 R5.1
N$12  (via drill 0.6)
  Top 0.254: v40.13,45.09 40.26,44.96 40.26,44.45 48.01,36.7 49.78,36.7 v50.8,35.69
  Bottom 0.762: LCD_LIME2.37 40.01,45.21 | 40.01,45.21 v40.13,45.09 | 40.01,45.21 LCD_LIME.37
  Bottom 1.016: v50.8,35.69 LCD_CON.37
N$13
  Bottom 0.254: 41.91,42.93 46.61,42.93 53.34,36.2
  Bottom 0.762: 41.91,42.93 41.27,42.93 LCD_LIME2.39 LCD_LIME.39
  Bottom 1.016: 53.34,36.2 LCD_CON.39
N$14  (via drill 0.6)
  Top 0.254: v13.84,36.96 14.61,36.96 18.67,41.02 18.67,45.09 20.57,46.99 20.57,49.28 v20.83,49.53
  Bottom 0.254: 20.95,38.35 20.57,37.97 14.86,37.97 v13.84,36.96 12.7,36.96 11.43,35.69 11.43,30.35 12.7,29.08
  Bottom 0.762: 20.95,38.35 LCD_LIME2.8 | v20.83,49.53 20.95,49.66 LCD_LIME.8
  Bottom 1.016: LCD_CON.8 12.7,29.08
N$15  (via drill 0.6)
  Top 0.254: v13.97,35.56 19.18,40.77 19.18,44.83 21.08,46.74 21.08,48.51 22.1,49.53 v22.23,49.53
  Bottom 0.254: 22.23,38.35 21.34,37.47 15.88,37.47 v13.97,35.56 13.97,30.35 15.24,29.08
  Bottom 0.762: 22.23,38.35 LCD_LIME2.10 | v22.23,49.53 LCD_LIME.10
  Bottom 1.016: LCD_CON.10 15.24,29.08
N$16  (via drill 0.6)
  Top 1.016: v44.96,4.19 44.96,9.65 44.32,10.29 v44.32,15.88
  Bottom 1.016: v44.32,15.88 44.2,16 44.2,17.64 T1.1 | EN/CTRL.2 44.2,3.43 v44.96,4.19
N$17  (via drill 0.6)
  Top 0.254: v19.05,35.56 21.21,37.72 21.21,43.81 24.64,47.24 24.64,49.4 v24.77,49.53
  Bottom 0.254: 24.77,38.35 22.86,36.45 19.94,36.45 v19.05,35.56 19.05,30.35 20.32,29.08
  Bottom 0.762: 24.77,38.35 LCD_LIME2.14 | v24.77,49.53 LCD_LIME.14
  Bottom 1.016: LCD_CON.14 20.32,29.08
N$18  (via drill 0.6)
  Top 0.254: v44.45,35.69 39.24,40.89 39.24,42.42 37.59,44.07 37.59,45.47 36.58,46.48 36.58,48.39 37.47,49.28 v37.47,49.4
  Bottom 0.254: 45.72,29.21 44.45,30.48 v44.45,35.69 43.18,36.96 39.62,36.96 38.99,37.59 38.35,37.59 37.47,38.48
  Bottom 0.762: v37.47,49.4 LCD_LIME.34 | 37.47,38.48 LCD_LIME2.34
  Bottom 1.016: LCD_CON.34 45.72,29.21
N$19
  Bottom 1.016: D1.3 39.41,20.07 39.75,20.07 41.27,21.59 R5.2
N$20  (via drill 0.6, 0.9)
  Top 1.016: 49.02,21.59 49.02,21.46 v49.4,21.46 v49.4,22.48
  Top 1.27: 49.02,21.59 49.02,28.57 44.32,33.27 7.62,33.27 7.24,33.66 | v6.22,34.67 7.24,33.66 | v6.22,34.67 v6.22,33.66 7.24,33.66 | 13.72,44.2 16,46.48 v16,46.74 | 13.72,44.2 v13.72,43.43 | v6.22,34.67 6.22,36.7 13.72,44.2
  Bottom 0.508: 16.76,43.43 LCD_LIME2.1 | 16.76,46.74 LCD_LIME.1
  Bottom 1.016: 5.08,33.66 5.08,34.67 v6.22,34.67 v6.22,33.66 5.08,33.66 | LCD_CON.1 5.08,33.66 | v49.4,21.46 49.4,21.97 | 49.4,21.97 49.02,21.97 | v49.4,22.48 49.4,21.97
  Bottom 1.27: v16,46.74 16.76,46.74 | v13.72,43.43 16.76,43.43
  Bottom 1.778: 49.02,21.97 PWR_JACK/5V_LCD_CON.3
N$21  (via drill 0.6)
  Top 0.254: v41.91,48.77 41.91,44.07 v48.01,37.97
  Bottom 0.254: 50.8,29.21 49.53,30.48 49.53,36.45 v48.01,37.97 40.51,37.97 40.01,38.48 | v41.91,48.77 41.15,49.53 40.51,49.53 40.01,50.04
  Bottom 0.762: 40.01,50.04 LCD_LIME.38 | 40.01,38.48 LCD_LIME2.38
  Bottom 1.016: 50.8,29.21 LCD_CON.38
N$22
  Bottom 1.778: PWR_JACK.1 49.91,14.1 49.91,15.49 50.29,15.11 | PWR_JACK/5V_LCD_CON.1 48.51,16.89 50.29,15.11 | 50.29,15.11 51.05,14.35
N$23  (via drill 0.6)
  Top 0.254: v49.02,38.86 47.88,38.86 42.8,43.94 v42.8,50.29
  Bottom 0.254: 53.34,29.21 52.07,30.48 52.07,35.81 v49.02,38.86 41.91,38.86
  Bottom 0.508: LCD_LIME2.40 41.27,38.86 41.53,38.86
  Bottom 0.762: v42.8,50.29 41.27,50.29 LCD_LIME.40 | 41.53,38.86 41.91,38.86
  Bottom 1.016: 53.34,29.21 LCD_CON.40
N$24  (via drill 0.6)
  Bottom 0.508: U1.5 3.94,10.41 3.94,9.91 3.94,9.65 3.94,9.46 U1.4
  Bottom 0.813: C7.1 3.05,9.91
  Bottom 1.016: 3.05,8.38 v3.43,8.38 3.94,8.38 | 3.05,8.38 C7.1 2.92,9.65 | 2.67,8.38 v2.41,8.38 v2.41,7.37 3.05,7.37 | 2.67,8.38 3.05,8.38 | 2.92,9.65 2.67,9.65 2.67,8.38 | 3.94,8.38 v4.45,8.38 v4.45,7.37 v3.43,7.37 3.05,7.37 | 2.92,9.65 3.94,9.65 3.94,8.38 | 3.05,7.37 R6.1 3.05,4.7
  Bottom 1.778: L1.2 3.05,16.46 C8.1 3.05,9.91 3.94,9.91
  other vias: 1.02,20.83 2.16,20.83 3.3,20.83
  pour Top (isolate 0.305): 3.94,22.23 0.51,22.23 0.51,6.73 4.95,6.73 4.95,9.02 3.94,9.02
  pour Bottom (isolate 0.305, no thermals): 0.51,22.23 4.06,22.23 4.06,13.59 0.51,13.59
N$123  (via drill 0.6)
  Bottom 0.508: U1.1 7.49,11.36 7.49,12.45
  Bottom 1.778: 7.49,12.45 7.49,16.33 L1.1 8.43,19.81 12.32,19.81 D2.2
  other vias: 6.22,11.56 6.22,12.57 8.51,12.83 8.51,13.84 7.11,20.83 8.26,20.83
  pour Top (isolate 0.305, no thermals): 6.6,22.23 6.6,13.34 6.22,12.95 5.84,12.95 5.84,11.05 10.41,11.05 10.41,22.23
  pour Bottom (isolate 0.305, no thermals): 10.54,21.84 10.54,21.08 14.35,21.08 14.35,17.14 10.54,17.14 10.54,11.18 5.84,11.18 5.84,13.08 6.35,13.08 6.6,13.34 6.6,21.84
N$126
  Bottom 0.508: U1.3 7.24,9.46 7.24,9.02 7.34,9.02 7.72,9.4
  Bottom 1.016: R11.1 R10.1 7.24,9.02
RXE0+  (via drill 0.5, 0.6)
  Top 0.508: v25.93,9.77 25.65,10.05 25.65,16.89 23.5,19.05 23.5,19.68 23.75,19.94 v23.75,20.07 | v22.86,35.56 22.86,36.04 24,37.19 24,43.31 v26.04,45.34
  Bottom 0.254: LCD.21 25.66,8.41 26.01,8.76
  Bottom 0.508: 26.01,8.76 26.01,9.69 v25.93,9.77 | v23.75,20.07 23.75,20.32 23.5,20.57 23.5,23.89 23.88,24.27 23.88,29.08 22.86,30.1
  Bottom 0.762: LCD_LIME.15 v26.04,45.34 LCD_LIME2.15
  Bottom 1.016: 22.86,30.1 LCD_CON.15 v22.86,35.56
RXE0-  (via drill 0.5, 0.6)
  Top 0.508: v25.09,9.02 25.02,9.09 25.02,16.62 22.86,18.78 22.86,19.68 22.61,19.94 v22.61,20.07 | v21.59,35.56 21.59,35.69 23.37,37.47 23.37,41.27 | v26.04,49.53 26.54,49.02 26.54,47.14 23.37,43.97 23.37,41.27 | 23.37,41.27 v22.99,41.27
  Bottom 0.254: LCD.20 25.16,8.64 25.15,8.64
  Bottom 0.508: v25.09,9.02 25.15,9.02 25.15,8.64 | v22.61,20.07 22.61,20.32 22.86,20.57 22.86,24.51 | 22.86,28.57 21.84,29.59 21.84,35.31 v21.59,35.56 | v22.99,41.27 23.24,41.27 23.62,40.89 25.4,40.89 26.04,40.26
  Bottom 0.762: 26.04,40.26 LCD_LIME2.16 | v26.04,49.53 LCD_LIME.16
  Bottom 1.016: 22.86,24.51 LCD_CON.16 22.86,28.57
RXE1+  (via drill 0.5, 0.6)
  Top 0.508: v28.07,11.81 27.8,12.08 27.8,18.95 26.04,20.71 26.04,21.72 26.29,21.97 v26.29,22.1 | v25.78,35.94 25.53,36.2 25.53,41.4 v25.91,41.78
  Bottom 0.254: LCD.24 27.16,8.63 27.3,8.78
  Bottom 0.508: 27.3,8.78 27.69,9.16 27.69,10.03 28.07,10.41 v28.07,11.81 | v26.29,22.1 26.16,22.23 26.16,22.48 26.04,22.61 26.04,23.89 26.42,24.27 26.42,29.21 25.4,30.23 | v25.91,41.78 26.54,41.78 27.3,42.55
  Bottom 0.762: LCD_LIME.17 LCD_LIME2.17 27.3,42.55
  Bottom 1.016: 25.4,30.23 LCD_CON.17 25.4,34.92 25.78,35.31 v25.78,35.94
RXE1-  (via drill 0.5, 0.6)
  Top 0.508: v27.15,11.06 27.15,18.69 25.4,20.45 25.4,21.72 25.15,21.97 v25.15,22.1 | v24.51,36.07 24.89,36.45 24.89,42.8 27.05,44.96 27.05,46.23 27.56,46.74 v27.56,48.39
  Bottom 0.254: LCD.23 26.66,8.86 | 26.66,8.86 26.8,8.99 26.8,9.14 | 26.79,9.16 26.8,9.16 26.8,9.14 | 26.66,8.86 26.66,9.14 26.8,9.14
  Bottom 0.508: 26.79,9.16 27.05,9.42 27.05,10.96 v27.15,11.06 | v25.15,22.1 25.15,22.35 25.4,22.61 25.4,24.51 | 25.4,28.7 24.38,29.72 24.38,35.94 v24.51,36.07 25.53,37.08 25.91,37.08 27.3,38.48 | v27.56,48.39 27.3,48.64 27.3,49.78
  Bottom 0.762: 27.3,38.48 LCD_LIME2.18 | 27.3,49.78 LCD_LIME.18
  Bottom 1.016: 25.4,24.51 LCD_CON.18 25.4,28.7
RXE2+  (via drill 0.5, 0.6)
  Top 0.508: v29.84,10.03 29.84,10.16 29.97,10.29 29.97,11.3 29.72,11.56 29.72,20.71 28.96,21.48 28.96,23.24 29.21,23.5 v29.21,23.88 | v27.94,35.69 27.94,37.08 27.56,37.47 27.56,43.28 28.57,44.3 28.57,44.7 v28.96,45.09
  Bottom 0.254: LCD.27 28.66,8.29 | 28.66,8.29 28.66,8.47 29.08,8.89 29.08,8.71 28.66,8.29
  Bottom 0.508: v29.84,10.03 29.84,9.91 29.08,9.14 29.08,8.89 | v29.21,23.88 29.21,24 28.96,24.26 28.96,29.34 27.94,30.35
  Bottom 0.762: 28.57,45.09 LCD_LIME.19 | v28.96,45.09 28.57,45.09 | 28.57,45.09 LCD_LIME2.19
  Bottom 1.016: 27.94,30.35 LCD_CON.19 v27.94,35.69
RXE2-  (via drill 0.5, 0.6)
  Top 0.508: v29.06,10.9 29.08,10.92 29.08,20.45 28.32,21.21 28.32,23.24 28.07,23.5 v28.07,23.88 | v26.92,36.58 26.92,43.56 27.94,44.58 27.94,45.47 28.57,46.1 v28.57,49.4
  Bottom 0.254: LCD.26 28.16,8.51 | 28.16,8.51 28.16,8.69 28.45,8.98 28.45,8.8 28.16,8.51
  Bottom 0.508: 28.45,8.98 28.45,9.53 28.93,10.01 28.93,10.77 v29.06,10.9 | 27.94,28.83 26.92,29.84 v26.92,36.58 28.57,38.23
  Bottom 0.762: LCD_CON.20 27.94,25.53 28.07,25.4 v28.07,23.88 | 28.57,38.23 LCD_LIME2.20 | v28.57,49.4 LCD_LIME.20
  Bottom 1.016: LCD_CON.20 27.94,28.83
RXEC+  (via drill 0.5, 0.6)
  Top 0.508: v30.25,6.1 30,6.35 28.96,6.35 28.7,6.1 28.69,6.1 27.8,5.21 25.65,5.21 24.13,6.73 24.13,14.49 21.08,17.54 21.08,18.17 21.34,18.43 v21.34,18.54 | v10.16,35.56 10.16,36.3 12.34,38.48 13.74,38.48 15.62,40.36 15.62,41.27 v16,41.66
  Bottom 0.254: LCD.30 30.16,6.19 v30.25,6.1 | v16,41.66 16.51,42.16 19.3,42.16 19.68,42.55
  Bottom 0.508: 10.16,30.48 11.18,29.46 11.18,24.62 11.8,24 20.19,24 21.08,23.11 21.08,19.05 21.34,18.8 v21.34,18.54
  Bottom 0.762: LCD_LIME.5 LCD_LIME2.5 19.68,42.55
  Bottom 1.016: 10.16,30.48 LCD_CON.5 v10.16,35.56
RXEC-  (via drill 0.5, 0.6)
  Top 0.508: v29.34,5.44 29.31,5.46 28.96,5.46 28.07,4.57 25.39,4.57 23.5,6.46 23.5,14.22 20.45,17.27 20.45,18.16 20.19,18.41 v20.19,18.54 | v19.56,49.53 19.3,49.53 18.67,48.9 18.67,46.74 14.99,43.05 14.99,40.77 | v8.89,35.56 8.89,35.94 12.06,39.12 13.46,39.12 14.99,40.64 14.99,40.77 | 14.99,40.77 v14.61,40.77
  Bottom 0.254: 29.34,6.3 29.66,6.62 29.66,6.69 | 29.66,6.69 LCD.29 | 29.66,6.69 29.34,6.37 29.34,6.22 | 19.68,40.26 19.3,40.64 14.73,40.64 v14.61,40.77
  Bottom 0.508: v29.34,5.44 29.34,6.22 29.34,6.3 | 10.16,24.74 11.53,23.37 19.93,23.37 20.45,22.85 20.45,19.05 20.19,18.8 v20.19,18.54 | 10.16,28.96 9.14,29.97 9.14,35.31 v8.89,35.56
  Bottom 0.762: 19.68,40.26 LCD_LIME2.6 | v19.56,49.53 19.68,49.66 LCD_LIME.6
  Bottom 1.016: 10.16,24.74 LCD_CON.6 10.16,28.96
VCC  (via drill 0.6, 0.8)
  Top 1.27: 32.13,2.92 35.56,2.92 41.66,9.02 v43.43,9.02 | 32.13,2.92 32.13,7.87 31.75,8.26 31.75,9.78 34.29,12.32 v34.29,15.62 | v19.56,14.48 19.56,7.87 24.51,2.92 32.13,2.92
  Bottom 0.254: LCD.2 16.16,8.79 16.26,8.89 | LCD.3 16.66,8.74 16.51,8.89 | LCD.4 17.16,8.37 16.64,8.89
  Bottom 0.508: 33.66,15.62 BKL_E.2 | FET2.3 44.53,9.02 43.94,9.02 | 44.58,7.24 3.3V/5.0V.1
  Bottom 1.016: v34.29,15.62 33.66,15.62 | 16.64,8.89 16.51,8.89 16.26,8.89 15.49,8.89 C2.1 C1.1 15.11,11.94 16.26,13.08 R7.1 R9.1 18.16,14.48 | R2.1 R1.2 18.16,16 18.16,14.48 | FET2.3 44.58,7.24 | 18.16,14.48 v19.56,14.48
  Bottom 1.27: 43.98,9.02 43.94,9.02 v43.43,9.02 v42.42,9.02
VLED_EN  (via drill 0.5, 0.6)
  Top 0.254: v18.92,3.68 17.78,4.83 17.27,4.83 15.75,6.35 15.75,10.67 17.14,12.06 v17.14,20.19 17.27,20.32 17.27,22.61 19.05,24.38 v19.05,25.27 | v23.75,48.26 23.75,47.12 20.7,44.07 20.7,38.48 v17.78,35.56
  Bottom 0.254: LCD.36 33.16,6.36 30.48,3.68 v18.92,3.68
  Bottom 0.508: v19.05,25.27 19.05,29.29 17.78,30.56
  Bottom 0.762: LCD_LIME2.11 LCD_LIME.11 23.5,48.01 v23.75,48.26
  Bottom 1.016: 17.78,30.56 LCD_CON.11 v17.78,35.56 | v17.14,20.19 17.14,19.05 R1.1
VPWM_EN  (via drill 0.6)
  Top 0.254: v17.4,3.94 17.27,3.94 15.24,5.97 15.24,10.92 15.88,11.56 v15.88,20.19 16.64,20.95 v16.64,25.27 | v23.5,49.53 22.86,48.9 22.86,46.99 20.19,44.32 20.19,39.24 v16.51,35.56
  Bottom 0.254: LCD.35 32.66,6.62 30.61,4.57 18.03,4.57 v17.4,3.94 | 17.78,29.08 16.51,30.35 v16.51,35.56 17.91,36.96 22.1,36.96 23.5,38.35
  Bottom 0.762: 23.5,38.35 LCD_LIME2.12 | v23.5,49.53 LCD_LIME.12
  Bottom 1.016: v16.64,25.27 17.78,25.27 LCD_CON.12 17.78,29.08 | v15.88,20.19 15.49,19.81 R2.2

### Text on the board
Top: Platkata trqbva da e debela 1mm!!!
Bottom: 60 errors
tNames: Platkata trqbva da e debela 1mm!!!
bNames: 39 | 1 | 2 | 5V_LCD_CON | https://www.olimex.com | PWR_JACK | A10-LCD15.6'' | 5V only | (C) 2014 | Rev.D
